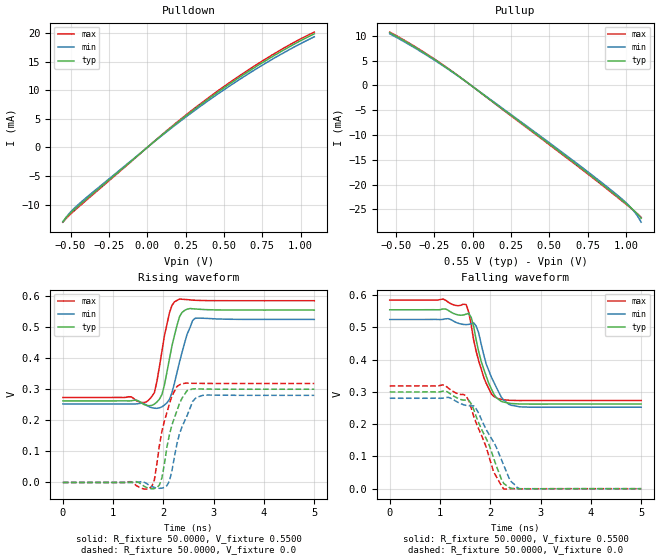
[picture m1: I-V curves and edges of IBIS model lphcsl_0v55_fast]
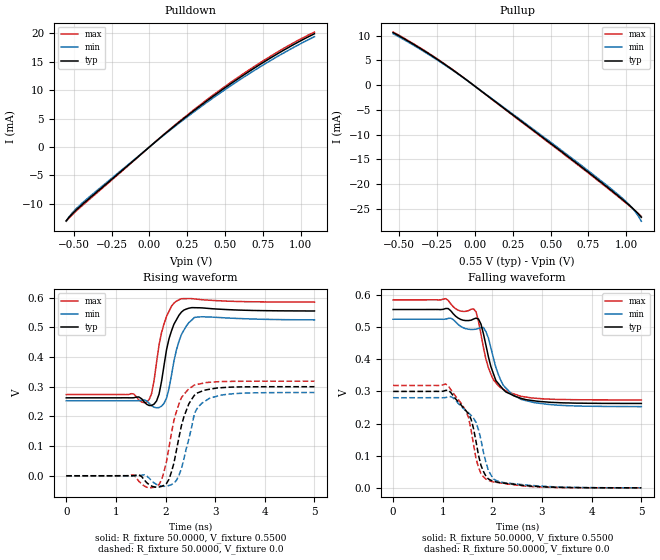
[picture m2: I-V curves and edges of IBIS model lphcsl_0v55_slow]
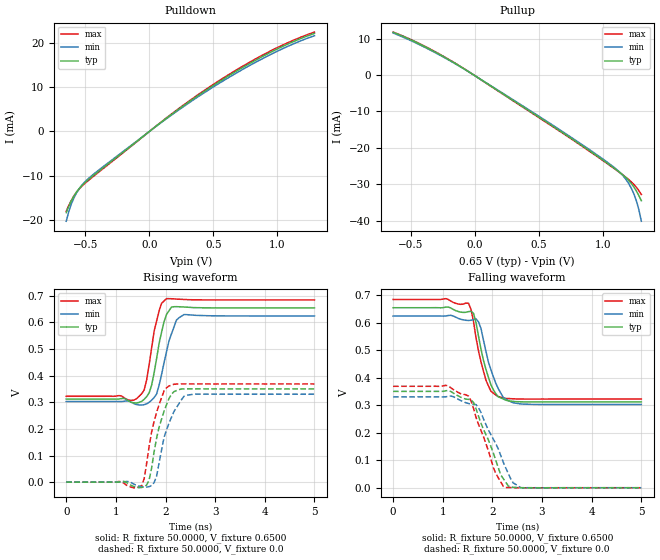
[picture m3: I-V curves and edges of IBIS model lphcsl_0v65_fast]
| Integrated Devices Technolgy, Inc
[IBIS Ver]   4.1
[File name]   9dbl0841b.ibs
[File Rev]   1.0
[Date]   May 16, 2016
[Source]   Integrated Devices Technolgy, Inc.
[Notes]   Rev 1.0 created by sg ; 05/16/2016
[Disclaimer] Integrated Device Technology, Inc. ("IDT") hereby grants the
   user of this ibis model a non-exclusive, nontransferable
   license to use this ibis model under the following terms. the
   user is granted this license only to use the ibis model and is
   not granted rights to sell, copy (except as needed to run the
   ibis model), rent, lease or sub-license the ibis model in
   whole or in part, or in modified form to anyone. the user may
   modify the ibis model to suit its specific applications, but
   rights to derivative works and such modifications shall belong
   to idt. this ibis model is provided on an as is" basis and idt
   makes absolutely no warranty with respect to the information
   contained herein. idt disclaims and customer waives all
   warranties, express and implied, including warranties of
   merchantability and fitness for a particular purpose. the
   entire risk as to quality and performance is with the user
   accordingly, in no event shall idt be liable for any direct or
   indirect damages, whether in contract or tort, including any
   lost profits or other incidental, consequential, exemplary, or
   punitive damages arising out of the use or application of the
   ibis model. further, idt reserves the right to make changes
   without notice to any product herein to improve reliability,
   function, or design. idt does not convey any license under
   patent rights or any other intellectual property rights,
   including those of third parties. idt is not obligated to
   provide maintenance or support for the licensed ibis model.
[Copyright]   Copyright 2012, Integrated Devices Technolgy, Inc. all rights
   reserved
[Component]   9dbl0841b
[Manufacturer] Integrated Device Technology, Inc.
[Package]
R_pkg   72.4655m   58.886m   86.045m
L_pkg   1.47175nH   1.11650nH   1.77850nH
C_pkg   0.07747pF   0.07444pF   0.08050pF
[Pin] signal_name  model_name
1   vSADR_tri   IN
2   ^vHIBW_BYPM_LOBW#   IN
3   FB_DNC   NC
4   FB_DNC#   NC
5   VDDR3.3   POWER
6   CLK_IN   IN
7   CLKIN#   IN
8   GNDR   GND
9   GNDDIG   GND
10   SCLK_3.3   SCIN
11   SDATA_3.3   SCIN
12   VDDDIG3.3   POWER
13   VDDIO   POWER
14   vOE0#   IN
15   DIF0   LP_HCSL
16   DIF0#   LP_HCSL
17   vOE1#   IN
18   DIF1   LP_HCSL
19   DIF1#   LP_HCSL
20   VDD3.3   POWER
21   VDDIO   POWER
22   GND   GND
23   DIF2   LP_HCSL
24   DIF2#   LP_HCSL
25   vOE2#   IN
26   DIF3   LP_HCSL
27   DIF3#   LP_HCSL
28   vOE3#   IN
29   GNDA   GND
30   VDDA3.3   POWER
31   VDDIO   POWER
32   DIF4   LP_HCSL
33   DIF4#   LP_HCSL
34   vOE4#   IN
35   DIF5   LP_HCSL
36   DIF5#   LP_HCSL
37   vOE5#   IN
38   VDD3.3   POWER
39   VDDIO   POWER
40   VSSPEX   GND
41   DIF6   LP_HCSL
42   DIF6#   LP_HCSL
43   vOE6#   IN
44   DIF7   LP_HCSL
45   DIF7#   LP_HCSL
46   vOE7#   IN
48   ^CKPWRGD_PD#   IN
49   ePAD   GND
[Diff Pin]  inv_pin  vdiff tdelay_typ tdelay_min  tdelay_max
15   16   NA   0   0   0
18   19   NA   0   0   0
23   24   NA   0   0   0
26   27   NA   0   0   0
32   33   NA   0   0   0
35   36   NA   0   0   0
41   42   NA   0   0   0
44   45   NA   0   0   0
[Model Selector] LP_HCSL
lphcsl_0v55_fast amplitude 0.55V, slew rate fast
lphcsl_0v55_slow amplitude 0.55V, slew rate slow
lphcsl_0v65_fast amplitude 0.65V, slew rate fast
lphcsl_0v65_slow amplitude 0.65V, slew rate slow
lphcsl_0v7_fast amplitude 0.7V, slew rate fast
lphcsl_0v7_slow amplitude 0.7V, slew rate slow
lphcsl_0v8_fast amplitude 0.8V, slew rate fast
lphcsl_0v8_slow amplitude 0.8V, slew rate slow
| Models and submodels in the file (10): lphcsl_0v55_fast (Output), lphcsl_0v55_slow (Output), lphcsl_0v65_fast (Output), lphcsl_0v65_slow (Output), lphcsl_0v7_fast (Output), lphcsl_0v7_slow (Output), lphcsl_0v8_fast (Output), lphcsl_0v8_slow (Output), SCIN (Input), IN (Input)
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|   Model lphcsl_0v55_fast
[Model]  lphcsl_0v55_fast
Model_type Output
Polarity   Non-Inverting
Vmeas =  0.4000V
Cref =   2.0000pF
Rref =   0.0
Vref =   0.4000V
C_comp   1.1000pF   1.0000pF   1.2000pF
[Temperature Range]   27.0000   70.0000   0.0
[Voltage Range]   0.5500V   0.5200V   0.5800V
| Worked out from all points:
|   slope of the pulldown table from 0 to 0.083 V, typ, clamps not added: 44.1 ohm
|   slope of the pullup table from 0 to 0.083 V, typ, clamps not added: 43 ohm
|   rising waveform, R_fixture 50.0000, V_fixture 0.5500: 20-80 % time 227ps typ, 259ps min, 207ps max; typ from 0.263 V to 0.555 V
|   rising waveform, R_fixture 50.0000, V_fixture 0.0: 20-80 % time 268ps typ, 304ps min, 250ps max; typ from 0 V to 0.3 V
|   falling waveform, R_fixture 50.0000, V_fixture 0.5500: 20-80 % time 309ps typ, 355ps min, 294ps max; typ from 0.555 V to 0.263 V
|   falling waveform, R_fixture 50.0000, V_fixture 0.0: 20-80 % time 464ps typ, 515ps min, 434ps max; typ from 0.3 V to 0 V
[Pulldown]
|Voltage   I(typ)   I(min)   I(max)
-550mV    -12.99mA   -13.03mA   -13.08mA
-530mV    -12.33mA   -12.26mA   -12.47mA
-490mV    -11.23mA   -11.02mA   -11.42mA
-390mV    -8.881mA   -8.62mA    -9.075mA
110mV     2.482mA    2.39mA     2.549mA
370mV     7.923mA    7.656mA    8.116mA
570mV     11.71mA    11.34mA    11.97mA
750mV     14.83mA    14.4mA     15.13mA
950mV     17.97mA    17.47mA    18.29mA
1.09V     19.91mA    19.39mA    20.21mA
[Pullup]
|Voltage   I(typ)   I(min)   I(max)
-540mV    10.63mA    10.41mA    10.74mA
-360mV    7.418mA    7.238mA    7.526mA
-160mV    3.369mA    3.276mA    3.432mA
-20mV     246.7uA    243.6uA    251.2uA
580mV     -13.63mA   -13.37mA   -13.79mA
840mV     -19.8mA    -19.51mA   -19.97mA
980mV     -23.27mA   -23.03mA   -23.41mA
1.04V     -24.85mA   -24.87mA   -24.93mA
1.08V     -26.06mA   -26.51mA   -26mA
1.1V      -26.77mA   -27.56mA   -26.57mA
[Ramp]
| variable   typ   min   max
dV/dt_r  0.1801/0.2684n   0.1683/0.3095n   0.1912/0.2502n
dV/dt_f  0.1754/0.3094n   0.1633/0.3555n   0.1869/0.2940n
R_load = 50.0000
[Rising Waveform]
R_fixture= 50.0000
V_fixture= 0.5500
V_fixture_min= 0.5200
V_fixture_max= 0.5800
|time   V(typ)   V(min)   V(max)
0s        262.6mV    252.7mV    273.6mV
1.46ns    265.2mV    252.9mV    263.5mV
1.67ns    247.8mV    248.3mV    260.3mV
1.82ns    252.1mV    239mV      289.2mV
1.97ns    283.2mV    243.4mV    422.4mV
2.12ns    398.1mV    267.2mV    546.2mV
2.32ns    533.6mV    387.7mV    590.4mV
2.47ns    557.8mV    476.9mV    588.7mV
2.63ns    558.5mV    528.4mV    586.5mV
5ns       555mV      524.8mV    585.1mV
[Rising Waveform]
R_fixture= 50.0000
V_fixture= 0.0
V_fixture_min= 0.0
V_fixture_max= 0.0
|time   V(typ)   V(min)   V(max)
0s        1.25uV     778nV      1.612uV
1.46ns    2.722mV    153uV      -10.02mV
1.77ns    -20.53mV   -13.19mV   -12.43mV
1.82ns    -19.75mV   -15.95mV   8.128mV
1.97ns    14.89mV    -18.28mV   164.5mV
2.12ns    154.4mV    4.72mV     253.3mV
2.32ns    254.5mV    157.2mV    314.4mV
2.58ns    301.1mV    260.7mV    319.2mV
2.78ns    300.7mV    280.3mV    318.9mV
5ns       300.1mV    280.5mV    318.6mV
[Falling Waveform]
R_fixture= 50.0000
V_fixture= 0.5500
V_fixture_min= 0.5200
V_fixture_max= 0.5800
|time   V(typ)   V(min)   V(max)
0s        555mV      524.8mV    585.1mV
1.52ns    541.3mV    508.9mV    571.1mV
1.62ns    531.5mV    511.9mV    507.6mV
1.72ns    460.7mV    504.3mV    425.5mV
1.87ns    370.9mV    415.3mV    345.5mV
2.02ns    309.7mV    346.7mV    294.3mV
2.17ns    276.5mV    298.8mV    278.6mV
2.37ns    265.4mV    261.6mV    274.2mV
2.58ns    262.7mV    254mV      273.4mV
5ns       262.6mV    252.7mV    273.6mV
[Falling Waveform]
R_fixture= 50.0000
V_fixture= 0.0
V_fixture_min= 0.0
V_fixture_max= 0.0
|time   V(typ)   V(min)   V(max)
0s        300.1mV    280.5mV    318.6mV
1.06ns    302.8mV    280.9mV    322.1mV
1.52ns    274.8mV    258.3mV    288mV
1.62ns    263.7mV    256.9mV    250.3mV
1.72ns    223.6mV    247.7mV    203.8mV
2.07ns    92.91mV    143.4mV    51.1mV
2.27ns    15.74mV    71.52mV    -1.457mV
2.42ns    864.6uV    21.19mV    -21.2uV
2.58ns    -99.14uV   -83.37uV   -356.3uV
5ns       1.577uV    575.4nV    1.592uV
|   Model lphcsl_0v55_slow
[Model]  lphcsl_0v55_slow
Model_type Output
Polarity   Non-Inverting
Vmeas =  0.4000V
Cref =   2.0000pF
Rref =   0.0
Vref =   0.4000V
C_comp   1.1000pF   1.0000pF   1.2000pF
[Temperature Range]   27.0000   70.0000   0.0
[Voltage Range]   0.5500V   0.5200V   0.5800V
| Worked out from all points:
|   slope of the pulldown table from 0 to 0.083 V, typ, clamps not added: 44.1 ohm
|   slope of the pullup table from 0 to 0.083 V, typ, clamps not added: 43 ohm
|   rising waveform, R_fixture 50.0000, V_fixture 0.5500: 20-80 % time 216ps typ, 224ps min, 210ps max; typ from 0.263 V to 0.555 V
|   rising waveform, R_fixture 50.0000, V_fixture 0.0: 20-80 % time 275ps typ, 259ps min, 264ps max; typ from 0 V to 0.3 V
|   falling waveform, R_fixture 50.0000, V_fixture 0.5500: 20-80 % time 347ps typ, 384ps min, 311ps max; typ from 0.555 V to 0.263 V
|   falling waveform, R_fixture 50.0000, V_fixture 0.0: 20-80 % time 329ps typ, 339ps min, 313ps max; typ from 0.3 V to 0 V
[Pulldown]
|Voltage   I(typ)   I(min)   I(max)
-550mV    -12.99mA   -13.03mA   -13.08mA
-530mV    -12.33mA   -12.26mA   -12.47mA
-490mV    -11.23mA   -11.02mA   -11.42mA
-390mV    -8.881mA   -8.62mA    -9.075mA
110mV     2.482mA    2.39mA     2.549mA
370mV     7.923mA    7.656mA    8.116mA
570mV     11.71mA    11.34mA    11.97mA
750mV     14.83mA    14.4mA     15.13mA
950mV     17.97mA    17.47mA    18.29mA
1.09V     19.91mA    19.39mA    20.21mA
[Pullup]
|Voltage   I(typ)   I(min)   I(max)
-540mV    10.63mA    10.41mA    10.74mA
-360mV    7.418mA    7.238mA    7.526mA
-160mV    3.369mA    3.276mA    3.432mA
-20mV     246.7uA    243.6uA    251.2uA
580mV     -13.63mA   -13.37mA   -13.79mA
840mV     -19.8mA    -19.51mA   -19.97mA
980mV     -23.27mA   -23.03mA   -23.41mA
1.04V     -24.85mA   -24.87mA   -24.93mA
1.08V     -26.06mA   -26.51mA   -26mA
1.1V      -26.77mA   -27.56mA   -26.57mA
[Ramp]
| variable   typ   min   max
dV/dt_r  0.1801/0.2751n   0.1683/0.2990n   0.1912/0.2641n
dV/dt_f  0.1754/0.3473n   0.1632/0.3841n   0.1869/0.3111n
R_load = 50.0000
[Rising Waveform]
R_fixture= 50.0000
V_fixture= 0.5500
V_fixture_min= 0.5200
V_fixture_max= 0.5800
|time   V(typ)   V(min)   V(max)
0s        262.6mV    252.7mV    273.6mV
1.31ns    262.5mV    252.8mV    276.6mV
1.62ns    240.9mV    252.1mV    248.3mV
1.72ns    236.9mV    236.1mV    277.1mV
1.82ns    252.2mV    229mV      383.4mV
1.97ns    372.2mV    244mV      512.1mV
2.12ns    488.1mV    338.9mV    571.5mV
2.32ns    551.5mV    475.7mV    596.8mV
2.63ns    566.2mV    534.5mV    595.1mV
5ns       555.3mV    525.3mV    585.2mV
[Rising Waveform]
R_fixture= 50.0000
V_fixture= 0.0
V_fixture_min= 0.0
V_fixture_max= 0.0
|time   V(typ)   V(min)   V(max)
0s        1.25uV     778nV      1.612uV
1.46ns    3.177mV    138.9uV    -18.33mV
1.82ns    -38.74mV   -29.22mV   -35.64mV
1.92ns    -35.82mV   -34.98mV   -13.98mV
2.07ns    -11.7mV    -32.74mV   96.17mV
2.22ns    86.17mV    -15.36mV   216.4mV
2.37ns    198.7mV    57.09mV    273.6mV
2.58ns    271mV      208.8mV    305.7mV
3.13ns    296.8mV    272.1mV    317.4mV
5ns       300.1mV    280.5mV    318.6mV
[Falling Waveform]
R_fixture= 50.0000
V_fixture= 0.5500
V_fixture_min= 0.5200
V_fixture_max= 0.5800
|time   V(typ)   V(min)   V(max)
0s        555mV      524.8mV    585.1mV
1.16ns    551.3mV    528mV      573mV
1.62ns    525.4mV    493.1mV    556.9mV
1.77ns    509.6mV    498.4mV    477.9mV
1.87ns    443.7mV    485.9mV    400.5mV
1.97ns    377.1mV    435.4mV    353.7mV
2.17ns    315.2mV    334mV      311.4mV
2.32ns    294.9mV    302.9mV    297.7mV
3.08ns    267.3mV    260.4mV    276.6mV
5ns       262.6mV    252.8mV    273.6mV
[Falling Waveform]
R_fixture= 50.0000
V_fixture= 0.0
V_fixture_min= 0.0
V_fixture_max= 0.0
|time   V(typ)   V(min)   V(max)
0s        300.1mV    280.5mV    318.6mV
1.11ns    303.6mV    283.1mV    317.5mV
1.52ns    230.2mV    233.4mV    218.5mV
1.57ns    213.9mV    225.7mV    180.6mV
1.67ns    144.2mV    203.9mV    90.84mV
1.77ns    69.8mV     149.6mV    44.43mV
1.92ns    27.5mV     54mV       23.24mV
2.02ns    20.78mV    27.76mV    18.26mV
2.37ns    12.28mV    13.7mV     10.74mV
5ns       29.12uV    81.62uV    12.5uV
|   Model lphcsl_0v65_fast
[Model]  lphcsl_0v65_fast
Model_type Output
Polarity   Non-Inverting
Vmeas =  0.4000V
Cref =   2.0000pF
Rref =   0.0
Vref =   0.4000V
C_comp   1.1000pF   1.0000pF   1.2000pF
[Temperature Range]   27.0000   70.0000   0.0
[Voltage Range]   0.6500V   0.6200V   0.6800V
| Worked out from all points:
|   slope of the pulldown table from 0 to 0.098 V, typ, clamps not added: 44.2 ohm
|   slope of the pullup table from 0 to 0.098 V, typ, clamps not added: 43.9 ohm
|   rising waveform, R_fixture 50.0000, V_fixture 0.6500: 20-80 % time 212ps typ, 252ps min, 200ps max; typ from 0.312 V to 0.655 V
|   rising waveform, R_fixture 50.0000, V_fixture 0.0: 20-80 % time 264ps typ, 304ps min, 255ps max; typ from 0 V to 0.35 V
|   falling waveform, R_fixture 50.0000, V_fixture 0.6500: 20-80 % time 274ps typ, 309ps min, 253ps max; typ from 0.655 V to 0.312 V
|   falling waveform, R_fixture 50.0000, V_fixture 0.0: 20-80 % time 440ps typ, 493ps min, 411ps max; typ from 0.35 V to 0 V
[Pulldown]
|Voltage   I(typ)   I(min)   I(max)
-650mV    -18.4mA    -20.35mA   -18.11mA
-630mV    -16.96mA   -18.14mA   -16.75mA
-610mV    -15.72mA   -16.43mA   -15.59mA
-590mV    -14.65mA   -15.06mA   -14.6mA
-550mV    -12.99mA   -13.03mA   -13.08mA
-510mV    -11.76mA   -11.6mA    -11.93mA
-410mV    -9.338mA   -9.072mA   -9.537mA
50mV      1.142mA    1.099mA    1.173mA
370mV     7.923mA    7.656mA    8.116mA
690mV     13.82mA    13.41mA    14.11mA
990mV     18.55mA    18.04mA    18.87mA
1.29V     22.21mA    21.69mA    22.52mA
[Pullup]
|Voltage   I(typ)   I(min)   I(max)
-640mV    11.75mA    11.55mA    11.82mA
-380mV    7.586mA    7.409mA    7.685mA
-120mV    2.462mA    2.392mA    2.508mA
640mV     -14.77mA   -14.51mA   -14.93mA
1.06V     -24.87mA   -24.62mA   -24.99mA
1.16V     -27.56mA   -27.79mA   -27.55mA
1.2V      -28.91mA   -29.73mA   -28.67mA
1.22V     -29.72mA   -30.99mA   -29.29mA
1.24V     -30.67mA   -32.51mA   -29.98mA
1.26V     -31.78mA   -34.42mA   -30.78mA
1.28V     -33.06mA   -36.87mA   -31.72mA
1.3V      -34.52mA   -40.17mA   -32.83mA
[Ramp]
| variable   typ   min   max
dV/dt_r  0.2102/0.2644n   0.1982/0.3040n   0.2213/0.2555n
dV/dt_f  0.2056/0.2744n   0.1930/0.3085n   0.2173/0.2534n
R_load = 50.0000
[Rising Waveform]
R_fixture= 50.0000
V_fixture= 0.6500
V_fixture_min= 0.6200
V_fixture_max= 0.6800
|time   V(typ)   V(min)   V(max)
0s        312mV      302.7mV    322.6mV
1.46ns    299.1mV    290mV      320.9mV
1.57ns    311.2mV    290.9mV    346.2mV
1.72ns    364.2mV    307.8mV    503.9mV
1.77ns    410.5mV    317.8mV    566.8mV
1.87ns    520.7mV    364mV      643.2mV
2.02ns    630.3mV    490.1mV    689.6mV
2.22ns    659.3mV    609mV      687.9mV
2.37ns    658.1mV    629.5mV    686.4mV
5ns       654.6mV    624.4mV    684.7mV
[Rising Waveform]
R_fixture= 50.0000
V_fixture= 0.0
V_fixture_min= 0.0
V_fixture_max= 0.0
|time   V(typ)   V(min)   V(max)
0s        795.8nV    0V         1.025uV
1.52ns    -20.29mV   -17.32mV   -13.12mV
1.57ns    -17.43mV   -18.81mV   12.71mV
1.67ns    8.433mV    -16.88mV   134.9mV
1.77ns    114.2mV    -2.001mV   228.1mV
1.97ns    266.6mV    167.8mV    342.7mV
2.07ns    314mV      222.1mV    361.2mV
2.32ns    350mV      309mV      369mV
2.47ns    350.6mV    327.9mV    369mV
5ns       350.3mV    330.4mV    368.9mV
[Falling Waveform]
R_fixture= 50.0000
V_fixture= 0.6500
V_fixture_min= 0.6200
V_fixture_max= 0.6800
|time   V(typ)   V(min)   V(max)
0s        654.6mV    624.4mV    684.7mV
1.52ns    640.4mV    608.3mV    670.8mV
1.62ns    633.9mV    611.2mV    603.9mV
1.72ns    551.2mV    603.3mV    497.8mV
1.87ns    430.5mV    495.8mV    391mV
1.97ns    374.6mV    429.8mV    351mV
2.12ns    330.7mV    359.6mV    331.3mV
2.27ns    318.5mV    322.1mV    324.9mV
2.58ns    312.5mV    304.4mV    322.6mV
5ns       312mV      302.7mV    322.6mV
[Falling Waveform]
R_fixture= 50.0000
V_fixture= 0.0
V_fixture_min= 0.0
V_fixture_max= 0.0
|time   V(typ)   V(min)   V(max)
0s        350.3mV    330.4mV    368.9mV
1.06ns    352.7mV    330.7mV    372.4mV
1.52ns    321.3mV    306.2mV    333.5mV
1.62ns    309.9mV    303.2mV    288.4mV
1.72ns    260.2mV    291mV      230.6mV
2.07ns    98.7mV     159.7mV    51.26mV
2.27ns    19.73mV    71.23mV    1.085mV
2.42ns    1.711mV    17.27mV    100.9uV
2.58ns    -45.42uV   62.27uV    -338uV
5ns       1.038uV    0V         1.14uV
